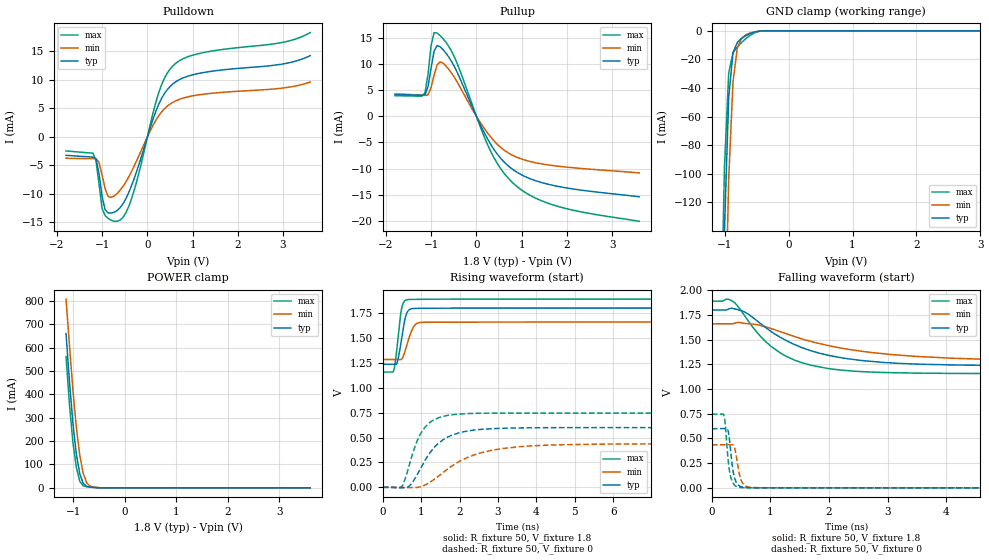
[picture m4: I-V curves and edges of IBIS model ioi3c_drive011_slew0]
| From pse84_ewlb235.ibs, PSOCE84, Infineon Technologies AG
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[Model] ioi3c_drive011_slew0
Model_type I/O
Enable   Active-High
Vinl  =  0.54
Vinh  =  1.26
Vmeas =  0.9
Cref  =  15e-12
| Capacitance   typ   min   max
C_comp   9.12545e-13 8.87504e-13 9.42456e-13
| Variables   typ   min   max
[GND Clamp Reference]   0   0   0
[POWER Clamp Reference]   1.8   1.66   1.89
[Pulldown Reference]   0   0   0
[Pullup Reference]   1.8   1.66   1.89
[Temperature Range]   25   125   -40
[Voltage Range]   1.8   1.66   1.89
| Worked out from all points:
|   slope of the pulldown table from 0 to 0.27 V, typ, clamps not added: 44.8 ohm
|   slope of the pullup table from 0 to 0.27 V, typ, clamps not added: 57.7 ohm
|   GND clamp passes 1 mA (typ) near -0.55 V on its own axis
|   POWER clamp passes 1 mA (typ) near -0.54 V on its own axis
|   falling waveform, R_fixture 50, V_fixture 1.8: 20-80 % time 1.16ns typ, 1.76ns min, 816ps max; typ from 1.8 V to 1.24 V
|   falling waveform, R_fixture 50, V_fixture 0: 20-80 % time 76.3ps typ, 85ps min, 71.8ps max; typ from 0.599 V to 0 V
|   rising waveform, R_fixture 50, V_fixture 1.8: 20-80 % time 148ps typ, 193ps min, 126ps max; typ from 1.24 V to 1.8 V
|   rising waveform, R_fixture 50, V_fixture 0: 20-80 % time 692ps typ, 1.22ns min, 452ps max; typ from 0 V to 0.599 V
[GND Clamp]
| Voltage   I(typ)   I(min)   I(max)
-1.204V   -737.9mA   -831.5mA   -678.7mA
-1.07V    -303.2mA   -410.8mA   -239.8mA
-1.003V   -139.9mA   -232.2mA   -95.74mA
-936.6mV  -46.51mA   -103.5mA   -29.5mA
-869.7mV  -15.31mA   -35.88mA   -15.36mA
-802.8mV  -8.166mA   -12.13mA   -11.29mA
-735.9mV  -5.335mA   -5.292mA   -8.195mA
-669mV    -3.356mA   -2.85mA    -5.457mA
-535.2mV  -837.9uA   -772uA     -1.483mA
-401.4mV  -47.36uA   -84.85uA   -76.77uA
3.6V      0A         0A         0A
[POWER Clamp]
| Voltage   I(typ)   I(min)   I(max)
-1.137V   660mA      807.5mA    561.8mA
-1.07V    454.5mA    608.2mA    356.2mA
-1.003V   275.7mA    418.4mA    193.6mA
-936.6mV  143.5mA    257.2mA    86.91mA
-869.7mV  59.43mA    137.9mA    27.31mA
-802.8mV  18.8mA     60.93mA    8.704mA
-735.9mV  6.231mA    21.35mA    5.155mA
-669mV    3.127mA    6.887mA    3.44mA
-535.2mV  940.9uA    1.232mA    1.058mA
-334.5mV  16.1uA     59.03uA    7.686uA
3.6V      0A         0A         0A
[Pulldown]
| Voltage   I(typ)   I(min)   I(max)
-1.8V     -3.256mA   -3.767mA   -2.48mA
-1.204V   -3.562mA   -3.839mA   -2.873mA
-1.137V   -3.887mA   -3.84mA    -4.196mA
-1.003V   -10.42mA   -6.637mA   -12.57mA
-936.6mV  -12.81mA   -9.105mA   -13.83mA
-869.7mV  -13.35mA   -10.45mA   -14.33mA
-602.1mV  -12.44mA   -9.384mA   -14.62mA
-334.5mV  -8.239mA   -5.816mA   -10.47mA
248.3mV   5.671mA    3.669mA    7.698mA
558.6mV   9.256mA    6.034mA    12.42mA
1.117V    11.1mA     7.344mA    14.57mA
3.6V      14.25mA    9.618mA    18.3mA
[Pullup]
| Voltage   I(typ)   I(min)   I(max)
-1.8V     4.157mA    4.308mA    3.943mA
-1.137V   4.15mA     4.01mA     4.534mA
-1.07V    5.698mA    4.112mA    8.074mA
-1.003V   9.236mA    5.498mA    13.51mA
-936.6mV  12.47mA    7.86mA     16.03mA
-869.7mV  13.54mA    9.82mA     15.93mA
-735.9mV  12.74mA    10.17mA    14.84mA
-468.3mV  9.185mA    7.186mA    11mA
310.3mV   -5.289mA   -3.904mA   -6.611mA
806.9mV   -10.18mA   -7.487mA   -12.75mA
1.738V    -13.29mA   -9.468mA   -17.06mA
3.6V      -15.39mA   -10.83mA   -20.08mA
[Ramp]
dV/dt_r   0.359394/0.692009n  0.261568/1.21721n  0.447321/0.452372n
dV/dt_f   0.338346/1.16025n  0.225657/1.76112n  0.439449/0.815614n
R_load = 50
[Falling Waveform]
R_fixture = 50
V_fixture = 1.8
V_fixture_min = 1.66
V_fixture_max = 1.89
| Time   V(typ)   V(min)   V(max)
0s        1.8V       1.66V      1.89V
356.3ps   1.817V     1.661V     1.889V
602ps     1.766V     1.663V     1.705V
1.007ns   1.585V     1.614V     1.434V
1.271ns   1.491V     1.559V     1.331V
1.701ns   1.387V     1.481V     1.24V
2.244ns   1.314V     1.411V     1.191V
2.939ns   1.269V     1.357V     1.168V
5.278ns   1.238V     1.295V     1.157V
800ns     1.236V     1.284V     1.158V
[Falling Waveform]
R_fixture = 50
V_fixture = 0
V_fixture_min = 0
V_fixture_max = 0
| Time   V(typ)   V(min)   V(max)
0s        599mV      435.9mV    745.5mV
206.4ps   598.9mV    435.9mV    733.1mV
230.7ps   598.8mV    435.9mV    629.3mV
267.1ps   593.5mV    435.9mV    347.6mV
297.6ps   503.2mV    435.8mV    182.5mV
383.6ps   108.4mV    412.3mV    28.91mV
475.9ps   17.12mV    121.9mV    4.276mV
546.6ps   4.634mV    31.46mV    1.937mV
1.071ns   782.6uV    928.9uV    563.7uV
800ns     13.01nV    842.7nV    5.03nV
[Rising Waveform]
R_fixture = 50
V_fixture = 1.8
V_fixture_min = 1.66
V_fixture_max = 1.89
| Time   V(typ)   V(min)   V(max)
0s        1.236V     1.284V     1.158V
285.4ps   1.236V     1.284V     1.176V
328.9ps   1.235V     1.284V     1.271V
386.4ps   1.271V     1.284V     1.47V
468.7ps   1.447V     1.282V     1.751V
551.8ps   1.644V     1.336V     1.865V
651.4ps   1.77V      1.462V     1.885V
844.5ps   1.797V     1.634V     1.888V
1.482ns   1.799V     1.659V     1.89V
800ns     1.8V       1.66V      1.89V
[Rising Waveform]
R_fixture = 50
V_fixture = 0
V_fixture_min = 0
V_fixture_max = 0
| Time   V(typ)   V(min)   V(max)
0s        13.01nV    842.5nV    5.03nV
499.2ps   -4.143mV   -1.203mV   11.63mV
682.6ps   10.63mV    -2.981mV   216.4mV
892.8ps   126.6mV    -1.288mV   466mV
1.223ns   345mV      49.94mV    651mV
1.635ns   493.8mV    168.6mV    718.1mV
2.201ns   565.5mV    299mV      740.6mV
3.569ns   596.5mV    408.2mV    745.7mV
5.499ns   599.4mV    432.8mV    745.6mV
50ns      599mV      435.9mV    745.5mV
